(* Logix 5000 DataType export A1000_IN; software revision 20.05 *)

TYPE A1000_STATUS :
STRUCT
   SystemReady : BOOL;
   reserved_0_1 : BOOL;
   reserved_0_2 : BOOL;
   reserved_0_3 : BOOL;
   reserved_0_4 : BOOL;
   reserved_0_5 : BOOL;
   ProcessingEnabled : BOOL;
   RunMode : BOOL;
   reserved_1_0 : BOOL;
   reserved_1_1 : BOOL;
   reserved_1_2 : BOOL;
   reserved_1_3 : BOOL;
   CommandExecuting : BOOL;
   CommandCompleted : BOOL;
   CommandFailed : BOOL;
   Error : BOOL;
   CommandResultCode : INT;
   ErrorID : INT;
   SoftEventAck0 : BOOL;
   SoftEventAck1 : BOOL;
   SoftEventAck2 : BOOL;
   SoftEventAck3 : BOOL;
   SoftEventAck4 : BOOL;
   SoftEventAck5 : BOOL;
   SoftEventAck6 : BOOL;
   SoftEventAck7 : BOOL;
   SoftEventAck8 : BOOL;
   SoftEventAck9 : BOOL;
   SoftEventAck10 : BOOL;
   SoftEventAck11 : BOOL;
   SoftEventAck12 : BOOL;
   SoftEventAck13 : BOOL;
   SoftEventAck14 : BOOL;
   SoftEventAck15 : BOOL;
   SoftEventAck16 : BOOL;
   SoftEventAck17 : BOOL;
   SoftEventAck18 : BOOL;
   SoftEventAck19 : BOOL;
   SoftEventAck20 : BOOL;
   SoftEventAck21 : BOOL;
   SoftEventAck22 : BOOL;
   SoftEventAck23 : BOOL;
   SoftEventAck24 : BOOL;
   SoftEventAck25 : BOOL;
   SoftEventAck26 : BOOL;
   SoftEventAck27 : BOOL;
   SoftEventAck28 : BOOL;
   SoftEventAck29 : BOOL;
   SoftEventAck30 : BOOL;
   SoftEventAck31 : BOOL;
   TriggerReady0 : BOOL;
   TriggerAck0 : BOOL;
   AcqError0 : BOOL;
   ExposureCompleted0 : BOOL;
   InspectionCompleted0 : BOOL;
   ResultsValid0 : BOOL;
   InspectionPassed0 : BOOL;
   ResultsBufferOverrun0 : BOOL;
   SetUserDataAck0 : BOOL;
   reserved_17_1 : BOOL;
   reserved_17_2 : BOOL;
   reserved_17_3 : BOOL;
   reserved_17_4 : BOOL;
   reserved_17_5 : BOOL;
   reserved_17_6 : BOOL;
   reserved_17_7 : BOOL;
   AcquiredImageID0 : INT;
   InspectedImageID0 : INT;
   InspectionResultCode0 : INT;
   TriggerReady1 : BOOL;
   TriggerAck1 : BOOL;
   AcqError1 : BOOL;
   ExposureCompleted1 : BOOL;
   InspectionCompleted1 : BOOL;
   ResultsValid1 : BOOL;
   InspectionPassed1 : BOOL;
   ResultsBufferOverrun1 : BOOL;
   SetUserDataAck1 : BOOL;
   reserved_25_1 : BOOL;
   reserved_25_2 : BOOL;
   reserved_25_3 : BOOL;
   reserved_25_4 : BOOL;
   reserved_25_5 : BOOL;
   reserved_25_6 : BOOL;
   reserved_25_7 : BOOL;
   TriggerReady2 : BOOL;
   TriggerAck2 : BOOL;
   AcqError2 : BOOL;
   ExposureCompleted2 : BOOL;
   InspectionCompleted2 : BOOL;
   ResultsValid2 : BOOL;
   InspectionPassed2 : BOOL;
   ResultsBufferOverrun2 : BOOL;
   SetUserDataAck2 : BOOL;
   reserved_33_1 : BOOL;
   reserved_33_2 : BOOL;
   reserved_33_3 : BOOL;
   reserved_33_4 : BOOL;
   reserved_33_5 : BOOL;
   reserved_33_6 : BOOL;
   reserved_33_7 : BOOL;
   TriggerReady3 : BOOL;
   TriggerAck3 : BOOL;
   AcqError3 : BOOL;
   ExposureCompleted3 : BOOL;
   InspectionCompleted3 : BOOL;
   ResultsValid3 : BOOL;
   InspectionPassed3 : BOOL;
   ResultsBufferOverrun3 : BOOL;
   SetUserDataAck3 : BOOL;
   reserved_41_1 : BOOL;
   reserved_41_2 : BOOL;
   reserved_41_3 : BOOL;
   reserved_41_4 : BOOL;
   reserved_41_5 : BOOL;
   reserved_41_6 : BOOL;
   reserved_41_7 : BOOL;
END_STRUCT
END_TYPE

TYPE A1000_IN :
STRUCT
   Status : A1000_STATUS;
   InspectionResults : SINT[452];
END_STRUCT
END_TYPE
